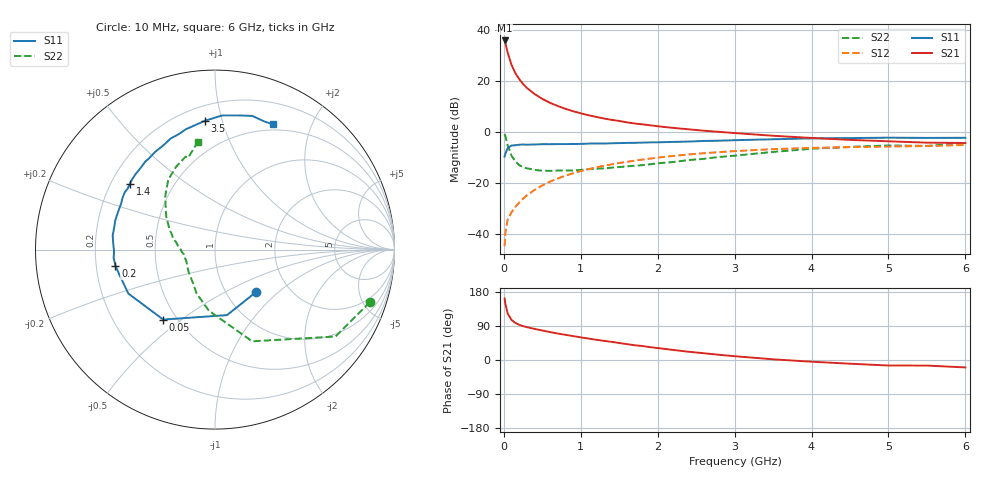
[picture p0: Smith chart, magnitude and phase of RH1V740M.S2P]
! SIEMENS Small Signal Semiconductors
! BFR106
! Si NPN RF Bipolar Junction Transistor in SOT23
! VCE = 1.75 V  IC = 40 mA
! Common Emitter S-Parameters:  August  1996
# GHz  S  MA  R  50
!  f  S11  S21  S12  S22
! GHz  MAG  ANG  MAG  ANG  MAG  ANG  MAG  ANG
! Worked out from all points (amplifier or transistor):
!   36 points, 10 MHz to 6 GHz, reference 50 ohm
!   highest |S21| = 36.0 dB at 10 MHz (marker M1)
!   |S21| within 3 dB of that: start of sweep to 35.83 MHz
!   unconditionally stable (mu >= 1): 248.5 MHz to 2.831 GHz; 5.077 GHz to end of sweep
!   at 250 MHz: K = 1.00, MAG = 22.3 dB, |S12| = -26.2 dB
!   at 1.4 GHz: K = 1.07, MAG = 7.2 dB, |S12| = -12.7 dB
!   at 6 GHz: K = 1.01, MAG = -0.2 dB, |S12| = -5.1 dB
!   S11 on the Smith chart (normalised r, x): 10 MHz: 1.37, -0.73; 50 MHz: 0.42, -0.43; 200 MHz: 0.28, -0.07; 1.4 GHz: 0.28, +0.32; 3.5 GHz: 0.30, +0.88; 6 GHz: 0.43, +1.48
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0.01  0.3289 -46.1  62.95 162.3  0.0057 78.2  0.9116 -18.7
0.02  0.3711 -79.6  56.19 148.2  0.0105 65.5  0.8279 -35.8
0.05  0.485 -126.5  36.21 122.6  0.0191 57.0  0.5511 -68.0
0.1  0.5413 -153.1  20.88 105.7  0.0265 57.3  0.342 -95.7
0.15  0.5502 -164.9  14.34 97.7  0.0337 60.4  0.2657 -112.6
0.2  0.5619 -170.8  10.95 93.0  0.0411 63.9  0.2238 -123.0
0.25  0.5667 -175.4  8.771 89.3  0.0488 66.1  0.2027 -132.8
0.3  0.5624 -178.6  7.34 86.7  0.0569 67.6  0.1934 -139.1
0.4  0.5688 176.0  5.569 82.0  0.0728 69.0  0.1799 -149.2
0.5  0.5755 172.1  4.471 77.8  0.089 69.2  0.1732 -156.2
0.6  0.5752 167.3  3.752 73.7  0.1058 68.6  0.1722 -160.5
0.7  0.5786 164.0  3.246 69.8  0.1218 67.8  0.1744 -164.5
0.9  0.5798 157.4  2.562 63.1  0.1542 65.4  0.1755 -171.8
1.1  0.5905 150.7  2.136 56.6  0.1857 62.7  0.1856 -175.9
1.4  0.5996 142.2  1.731 47.9  0.231 57.8  0.1987 177.2
1.7  0.6131 133.8  1.471 39.0  0.2729 53.0  0.2174 170.3
2.2  0.6383 121.5  1.204 26.6  0.3382 44.5  0.2569 160.0
2.8  0.6741 107.5  1.006 13.7  0.402 34.5  0.323 146.9
3.5  0.7199 94.5  0.843 1.8  0.4599 23.5  0.4054 133.2
4.5  0.7588 80.2  0.7 -9.8  0.5036 9.3  0.5099 115.2
5.5  0.765 68.9  0.617 -14.7  0.5295 0.7  0.5333 106.3
6  0.7693 65.0  0.608 -19.6  0.5553 -6.1  0.6057 99.2
